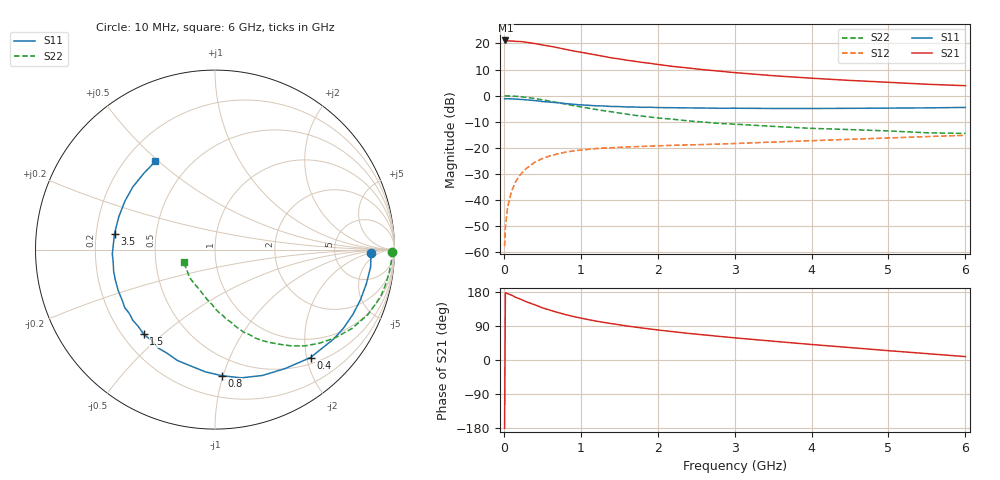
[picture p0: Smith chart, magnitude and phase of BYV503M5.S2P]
! SIEMENS Small Signal Semiconductors
! BFY420
! Si NPN RF SIEGET Grounded Emitter Transistor in MICRO-X
! VCE = 0.5 V  IC = 3.5 mA
! Common Emitter S-Parameters:  October  1996
# GHz  S  MA  R  50
!  f  S11  S21  S12  S22
! GHz  MAG  ANG  MAG  ANG  MAG  ANG  MAG  ANG
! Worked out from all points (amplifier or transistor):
!   36 points, 10 MHz to 6 GHz, reference 50 ohm
!   highest |S21| = 21.1 dB at 20 MHz (marker M1)
!   |S21| within 3 dB of that: start of sweep to 736.7 MHz
!   unconditionally stable (mu >= 1): 3.332 GHz to end of sweep
!   at 250 MHz: K = 0.09, MSG = 24.9 dB, |S12| = -29.1 dB
!   at 1.4 GHz: K = 0.47, MSG = 17.2 dB, |S12| = -20.0 dB
!   at 6 GHz: K = 1.22, MAG = 6.7 dB, |S12| = -15.2 dB
!   S11 on the Smith chart (normalised r, x): 10 MHz: 14, -2; 400 MHz: 0.61, -2.07; 800 MHz: 0.36, -0.99; 1.5 GHz: 0.29, -0.43; 3.5 GHz: 0.28, +0.07; 6 GHz: 0.32, +0.49
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0.01  0.8672 -1.4  11.39 -179.9  0.0013 97.2  0.9872 -0.7
0.02  0.8697 -2.7  11.4 177.8  0.003 88.3  0.9828 -1.5
0.05  0.8724 -6.4  11.14 174.9  0.0074 85.3  0.9851 -3.9
0.1  0.8644 -12.8  11.16 171.3  0.0146 84.0  0.9778 -8.0
0.15  0.8576 -18.9  10.96 165.7  0.0219 78.5  0.9691 -12.0
0.25  0.839 -31.5  10.76 157.4  0.035 72.2  0.94 -19.6
0.3  0.8271 -37.2  10.47 153.1  0.041 69.6  0.9245 -23.2
0.4  0.803 -48.5  9.966 145.9  0.0527 63.0  0.8801 -30.0
0.5  0.7696 -59.4  9.344 137.8  0.062 57.4  0.8307 -36.2
0.6  0.7495 -69.3  8.843 131.5  0.07 52.9  0.7824 -41.8
0.8  0.7033 -87.0  7.711 120.0  0.0823 44.1  0.6881 -51.3
0.9  0.6829 -94.6  7.2 114.9  0.0868 41.3  0.6462 -55.0
1.1  0.6522 -108.8  6.393 106.5  0.0934 36.0  0.5735 -62.3
1.3  0.6329 -120.1  5.641 99.3  0.0991 32.0  0.5122 -67.8
1.5  0.6162 -130.1  5.047 93.1  0.1019 28.9  0.4626 -73.0
1.8  0.5954 -143.3  4.325 84.4  0.1061 25.8  0.4043 -78.9
2.2  0.5857 -157.0  3.621 74.7  0.1115 22.5  0.3517 -86.3
2.8  0.5714 -173.3  2.943 62.3  0.118 19.9  0.293 -95.8
3.5  0.5668 170.9  2.407 49.6  0.1287 17.6  0.2569 -105.2
4.5  0.5699 151.6  1.953 32.8  0.1453 13.5  0.223 -120.9
5.5  0.5814 132.9  1.649 16.8  0.1638 8.5  0.1936 -144.0
6  0.5934 124.0  1.548 9.0  0.1733 5.8  0.1885 -157.6
